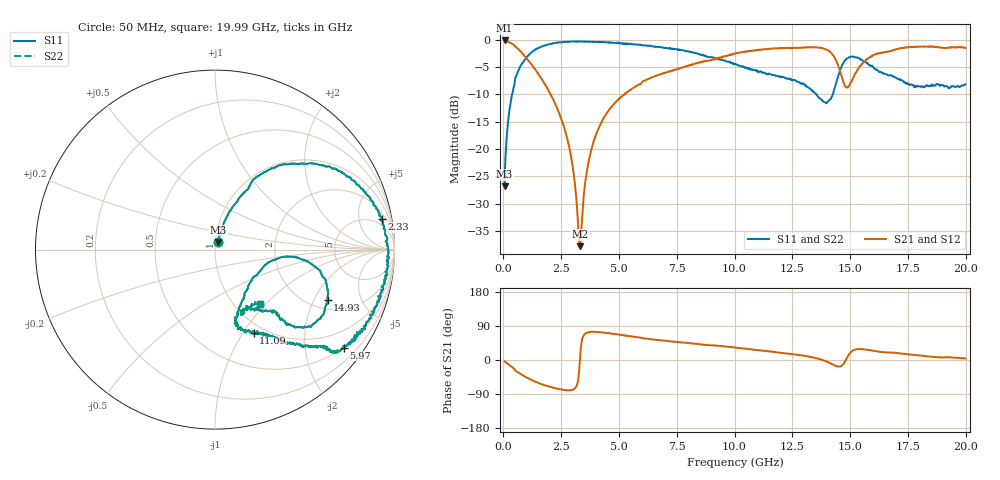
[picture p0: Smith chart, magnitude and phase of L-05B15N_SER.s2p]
! Data Taken on a HP 8720C VNA using a series-through fixture with TRL* de-embedding
#	mhz	s	ma	r	50
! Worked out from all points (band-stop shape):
!   998 points, 50 MHz to 19.99 GHz, reference 50 ohm
!   highest |S21| = -0.12 dB at 50 MHz (marker M1); lowest = -37.8 dB at 3.31 GHz (marker M2)
!   |S21| within 3 dB of the highest: 9.501 GHz to 14.31 GHz (4.812 GHz wide, 40.4 % of centre); 15.86 GHz to end of sweep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
!   lowest |S11| = -26.9 dB at 50 MHz (marker M3), VSWR 1.10, Z = 51.6 + j4.32 ohm
!   |S11| at or under -10 dB: start of sweep to 374.2 MHz; 13.55 GHz to 14.25 GHz (699.5 MHz wide, 5.03 % of centre)
!   |S22| runs from -26.9 to -0.3 dB; largest |S21 - S12| = 0
!   S11 on the Smith chart (normalised r, x): 50 MHz: 1.03, +0.09; 2.33 GHz: 3, +10; 5.97 GHz: 0.49, -2.89; 11.09 GHz: 0.88, -1.12; 14.93 GHz: 2.45, -2.58; 19.99 GHz: 1.30, -0.92
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50  0.04542 67.0  0.986 -3.8  0.986 -3.8  0.04542 67.0
250  0.2189 69.4  0.9501 -13.1  0.9501 -13.1  0.2189 69.4
610  0.5016 58.1  0.8335 -31.4  0.8335 -31.4  0.5016 58.1
1270  0.7873 36.2  0.5744 -54.0  0.5744 -54.0  0.7873 36.2
2330  0.944 10.5  0.2347 -75.7  0.2347 -75.7  0.944 10.5
2910  0.9643 0.9  0.08912 -79.7  0.08912 -79.7  0.9643 0.9
3310  0.9612 -5.0  0.01289 1.5  0.01289 1.5  0.9612 -5.0
3390  0.9622 -6.3  0.02181 50.0  0.02181 50.0  0.9622 -6.3
3650  0.9661 -9.5  0.07012 72.9  0.07012 72.9  0.9661 -9.5
4090  0.9581 -15.6  0.1502 73.7  0.1502 73.7  0.9581 -15.6
5970  0.9015 -37.3  0.4011 58.5  0.4011 58.5  0.9015 -37.3
6710  0.8598 -41.1  0.4773 52.6  0.4773 52.6  0.8598 -41.1
10030  0.6018 -55.2  0.7512 33.1  0.7512 33.1  0.6018 -55.2
11090  0.513 -65.2  0.8081 25.4  0.8081 25.4  0.513 -65.2
13350  0.3421 -65.9  0.8546 6.9  0.8546 6.9  0.3421 -65.9
13990  0.2631 -35.3  0.8096 -4.3  0.8096 -4.3  0.2631 -35.3
14410  0.4091 -5.5  0.6351 -16.3  0.6351 -16.3  0.4091 -5.5
14930  0.6869 -23.9  0.3746 12.3  0.3746 12.3  0.6869 -23.9
15510  0.6542 -41.7  0.6028 28.5  0.6028 28.5  0.6542 -41.7
16670  0.4697 -46.4  0.7803 19.9  0.7803 19.9  0.4697 -46.4
18230  0.3688 -66.8  0.8628 10.3  0.8628 10.3  0.3688 -66.8
19990  0.3913 -50.2  0.842 4.0  0.842 4.0  0.3913 -50.2
